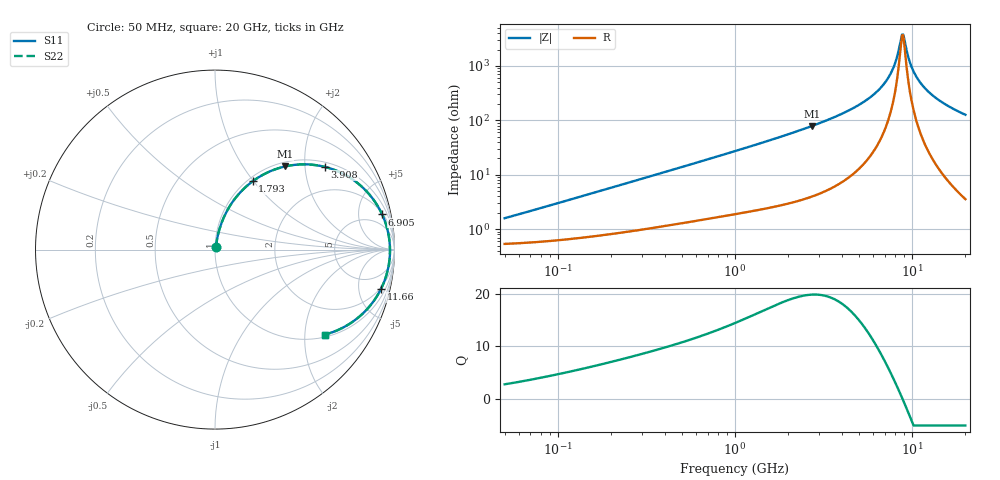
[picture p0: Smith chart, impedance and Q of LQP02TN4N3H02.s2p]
!Murata Part Number: LQP02TN4N3H02
!These Parameters are Measured in Series Mode Connection
!  o--[Z]--o
!Port1  Port2
!  o-------o
!Freq. Start=50[MHz] Stop=20[GHz], 401[Steps]
# Hz S RI R 50
!Freq.(Hz) S11(Real) S11(Imag) S21(Real) S21(Imag) S12(Real) S12(Imag) S22(Real) S22(Imag)
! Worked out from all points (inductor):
!   401 points, 50 MHz to 20 GHz, reference 50 ohm
!   read as one part in series: L = 4.74 nH near 54.7 MHz
!   highest Q = 19.8 at 2.728 GHz (marker M1), where L = 4.61 nH
!   self-resonance near 8.775 GHz
!   S11 on the Smith chart (normalised r, x): 50 MHz: 1.01, +0.03; 1.793 GHz: 1.05, +0.99; 3.908 GHz: 1.14, +2.54; 6.905 GHz: 2.19, +9.09; 11.66 GHz: 1.80, -8.15; 20 GHz: 1.07, -2.53
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5e7  0.00555 0.0148  0.9944 -0.0148  0.9944 -0.0148  0.00555 0.0148
1.364002e8  0.00846 0.0391  0.9915 -0.0391  0.9915 -0.0391  0.00846 0.0391
3.721004e8  0.0212 0.1006  0.9788 -0.1006  0.9788 -0.1006  0.0212 0.1006
1e9  0.0836 0.2443  0.9164 -0.2443  0.9164 -0.2443  0.0836 0.2443
1.793498e9  0.2092 0.3801  0.7908 -0.3801  0.7908 -0.3801  0.2092 0.3801
2.728004e9  0.3906 0.4633  0.6094 -0.4633  0.6094 -0.4633  0.3906 0.4633
3.908127e9  0.6116 0.4609  0.3884 -0.4609  0.3884 -0.4609  0.6116 0.4609
5.433528e9  0.8207 0.3481  0.1793 -0.3481  0.1793 -0.3481  0.8207 0.3481
6.217679e9  0.8897 0.2687  0.1103 -0.2687  0.1103 -0.2687  0.8897 0.2687
6.905011e9  0.9312 0.1958  0.0688 -0.1958  0.0688 -0.1958  0.9312 0.1958
7.442007e9  0.953 0.1391  0.047 -0.1391  0.047 -0.1391  0.953 0.1391
8.020766e9  0.9676 0.0797  0.0324 -0.0797  0.0324 -0.0797  0.9676 0.0797
8.644534e9  0.9745 0.0186  0.0255 -0.0186  0.0255 -0.0186  0.9745 0.0186
8.774992e9  0.9749 0.00626  0.0251 -0.00626  0.0251 -0.00626  0.9749 0.00626
8.907419e9  0.975 -0.00607  0.025 0.00607  0.025 0.00607  0.975 -0.00607
9.041845e9  0.9748 -0.0184  0.0252 0.0184  0.0252 0.0184  0.9748 -0.0184
9.600142e9  0.9709 -0.0676  0.0291 0.0676  0.0291 0.0676  0.9709 -0.0676
1.004137e10  0.9647 -0.104  0.0353 0.104  0.0353 0.104  0.9647 -0.104
1.066139e10  0.9522 -0.1516  0.0478 0.1516  0.0478 0.1516  0.9522 -0.1516
1.166392e10  0.9247 -0.2195  0.0753 0.2195  0.0753 0.2195  0.9247 -0.2195
1.460232e10  0.8173 -0.362  0.1827 0.362  0.1827 0.362  0.8173 -0.362
2e10  0.6134 -0.4731  0.3866 0.4731  0.3866 0.4731  0.6134 -0.4731
